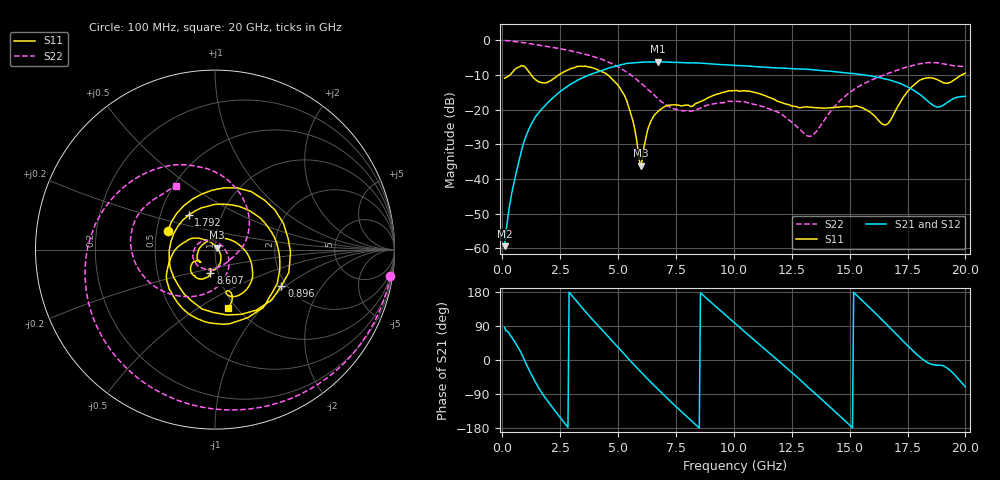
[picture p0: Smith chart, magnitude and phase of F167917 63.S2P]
!  2-Port S-parameters saved by WinCal
! VAR MeasName=S-Parameters (CALIBRATED_DATA) read from VNA (N5242A)
! VAR MeasDate=2016-11-22 9:03:09
! VAR NAME=F167917 63
! VAR FILENAME=F167917 63.S2P
! VAR DATE=2016-11-22 9:03:10
! VAR PHYS_PORTS=1,2
# Hz S DB R 50
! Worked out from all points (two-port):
!   401 points, 100 MHz to 20 GHz, reference 50 ohm
!   highest |S21| = -6.25 dB at 6.717 GHz (marker M1); lowest = -59.3 dB at 100 MHz (marker M2)
!   |S21| within 3 dB of the highest: 4.079 GHz to 14.59 GHz (10.51 GHz wide, 113 % of centre)
!   lowest |S11| = -36.2 dB at 5.971 GHz (marker M3), VSWR 1.03, Z = 51.1 + j1.15 ohm
!   |S11| at or under -10 dB: start of sweep to 338.5 MHz; 1.242 GHz to 2.449 GHz (1.207 GHz wide, 65.4 % of centre); 4.553 GHz to 19.85 GHz (15.29 GHz wide, 125 % of centre)
!   |S22| runs from -27.7 to -0.1 dB; largest |S21 - S12| = 0.0042
!   S11 on the Smith chart (normalised r, x): 100 MHz: 0.57, +0.13; 896 MHz: 1.88, -0.92; 1.792 GHz: 0.70, +0.28; 8.607 GHz: 0.92, -0.24; 20 GHz: 0.91, -0.67
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1e8  -10.96 158.2  -59.34 86.6  -59.80 87.7  -0.10 -8.7
4.98e8  -8.76 70.7  -41.35 51.9  -41.33 51.4  -0.36 -40.7
8.96e8  -7.51 -28.7  -30.23 8.5  -30.29 8.9  -0.72 -70.4
1.34375e9  -10.88 -135.7  -23.12 -48.1  -23.11 -47.8  -1.20 -100.2
1.7915e9  -12.33 127.5  -19.29 -94.5  -19.28 -94.4  -1.68 -126.5
2.63725e9  -9.23 6.0  -14.11 -162.6  -14.12 -162.3  -2.65 -169.4
3.43325e9  -7.56 -67.6  -10.94 138.9  -10.89 139.2  -3.83 154.9
4.32875e9  -9.19 -132.5  -8.71 78.1  -8.64 78.0  -5.62 115.7
5.075e9  -13.74 175.1  -7.18 28.5  -7.17 28.2  -7.95 81.1
5.5725e9  -21.66 137.6  -6.59 -5.3  -6.60 -5.5  -10.17 57.4
5.9705e9  -36.21 46.6  -6.38 -30.6  -6.39 -30.8  -12.28 37.9
6.71675e9  -20.58 -78.3  -6.25 -77.1  -6.25 -77.0  -16.86 1.3
6.7665e9  -20.35 -80.4  -6.25 -80.0  -6.25 -80.0  -17.16 -0.9
8.60725e9  -17.59 -101.1  -6.64 174.7  -6.63 174.8  -19.40 -88.8
1.005e10  -14.54 -123.9  -7.26 96.8  -7.25 96.9  -17.65 -148.6
1.17415e10  -17.05 -150.4  -7.97 7.2  -7.93 7.1  -20.26 158.1
1.338325e10  -19.40 -141.1  -8.51 -81.6  -8.48 -81.5  -27.50 39.6
1.507475e10  -19.26 -145.0  -9.56 -175.6  -9.56 -175.9  -14.73 -77.2
1.67165e10  -23.49 73.5  -11.45 86.8  -11.56 87.1  -9.46 -130.7
1.801e10  -11.61 -37.7  -15.55 9.4  -15.44 9.9  -6.85 -173.0
1.8806e10  -11.47 -73.7  -19.30 -13.8  -19.15 -13.0  -6.55 156.1
2e10  -9.51 -77.8  -16.19 -70.8  -16.03 -70.6  -7.60 121.4
